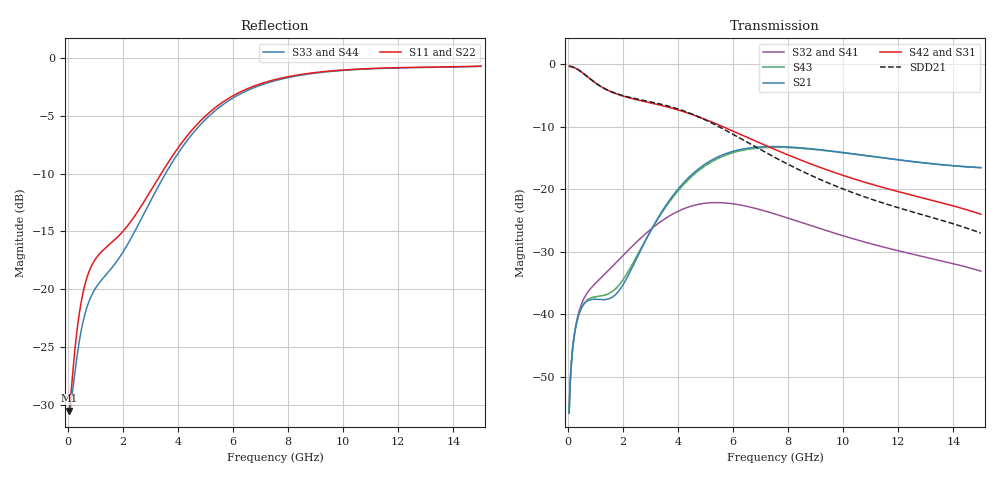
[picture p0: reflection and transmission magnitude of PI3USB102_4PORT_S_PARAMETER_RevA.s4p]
! NPort=4 DATA=800 NOISE=0 GROUPDELAY=0 COMPLEX_DATAFORMAT=POLAR
! NumOfBlock=1 NumOfParam=0
! .MODEL Smodel S TSTONEFILE=PI3USB102_4PORT_S_PARAMETER_RevA.s4p TYPE=S
!  -- The above .MODEL line can be used for the S element in the netlist.
! PORT DEFINITION
! PORT1 = INPUT+
! PORT2 = INPUT-
! PORT3 = OUTPUT+
! PORT4 = OUTPUT-
# Hz S MA R  50
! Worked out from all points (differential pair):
!   800 points, 50 MHz to 15 GHz, reference 50 ohm
!   strongest paths, dB at 50 MHz, 3.792 GHz, 7.534 GHz, 11.28 GHz, 15 GHz:
!     S42: -0.4, -7.1, -13.7, -19.5, -24.0
!     S31: -0.4, -7.1, -13.7, -19.5, -24.0
!     S21: -55.8, -21.2, -13.2, -14.9, -16.6
!     S43: -55.8, -21.4, -13.3, -14.9, -16.6
!     S32: -55.8, -24.0, -24.0, -29.0, -33.1
!     S41: -55.8, -24.0, -24.0, -29.0, -33.1
!   taken as a pair (ports 2,1 in; 4,3 out), SDD21 dB: -0.4, -6.9, -15.0, -22.0, -27.0
!   lowest |S11| = -30.5 dB at 50 MHz (marker M1), VSWR 1.06, Z = 52.8 - j1.33 ohm
!   |S11| at or under -10 dB: start of sweep to 3.391 GHz
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5e7  0.02975 -25.0  0.001627 84.6  0.9601 -2.9  0.001625 84.6
     0.001627 84.6  0.02976 -24.9  0.001625 84.6  0.9601 -2.9
     0.9601 -2.9  0.001625 84.6  0.02902 -19.9  0.001627 84.8
     0.001625 84.6  0.9601 -2.9  0.001627 84.8  0.02901 -19.9
2.93242e8  0.05979 -92.1  0.007996 66.4  0.9227 -16.3  0.00819 65.9
           0.007996 66.4  0.05979 -92.1  0.00819 65.9  0.9227 -16.3
           0.9227 -16.3  0.00819 65.9  0.04683 -83.9  0.008016 67.3
           0.00819 65.9  0.9227 -16.3  0.008016 67.3  0.04683 -83.9
7.42303e8  0.1165 -149.9  0.01292 51.1  0.7823 -35.8  0.01523 47.3
           0.01292 51.1  0.1165 -149.8  0.01523 47.3  0.7823 -35.8
           0.7823 -35.8  0.01523 47.3  0.08663 -147.7  0.01322 53.2
           0.01523 47.3  0.7823 -35.8  0.01322 53.2  0.08664 -147.7
3.06245e9  0.2728 51.1  0.04888 113.4  0.4857 -87.2  0.04883 11.1
           0.04888 113.4  0.2728 51.1  0.04883 11.1  0.4857 -87.2
           0.4857 -87.2  0.04883 11.1  0.2478 44.9  0.04853 109.0
           0.04883 11.1  0.4857 -87.2  0.04853 109.0  0.2478 44.9
5.21421e9  0.5912 -27.0  0.1703 72.7  0.345 -136.7  0.07805 -57.7
           0.1703 72.7  0.5912 -27.0  0.07805 -57.7  0.345 -136.7
           0.345 -136.7  0.07804 -57.7  0.5731 -28.7  0.1651 72.0
           0.07804 -57.7  0.345 -136.7  0.1651 72.0  0.573 -28.7
8.45119e9  0.8484 -86.3  0.2141 11.7  0.1713 167.2  0.05453 -144.3
           0.2141 11.7  0.8484 -86.3  0.05452 -144.3  0.1712 167.2
           0.1712 167.2  0.05452 -144.3  0.8423 -86.5  0.2122 12.0
           0.05452 -144.3  0.1713 167.2  0.2122 12.0  0.8423 -86.5
1.5e10  0.9223 -127.1  0.1487 -29.3  0.0631 75.0  0.02218 102.5
        0.1487 -29.3  0.9223 -127.1  0.02218 102.5  0.06309 75.0
        0.06309 75.0  0.02218 102.5  0.9211 -127.1  0.1485 -29.2
        0.02218 102.5  0.0631 75.0  0.1485 -29.2  0.9211 -127.1
